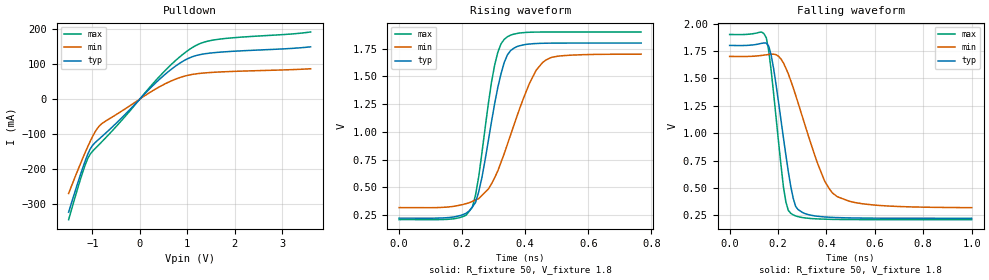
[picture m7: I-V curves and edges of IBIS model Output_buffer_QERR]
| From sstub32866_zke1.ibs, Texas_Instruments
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|   Model   Output_buffer_QERR
[Model]   Output_buffer_QERR
Model_type   Open_drain
Polarity   Non-Inverting
Vmeas  =   0.90
Cref   =   10.0p
Rref   =   1000
Vref   =   1.8
|Variable   typ   min   max
C_comp   1.120e-12   0.305e-12   1.791e-12
|Variable   typ   min   max
[Voltage range]   1.8   1.7   1.9
|Variable   typ   min   max
[Temperature range]  27   125   0.0
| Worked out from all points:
|   slope of the pulldown table from 0 to 0.27 V, typ, clamps not added: 7.15 ohm
|   rising waveform, R_fixture 50, V_fixture 1.8: 20-80 % time 61.3ps typ, 107ps min, 50.9ps max; typ from 0.223 V to 1.8 V
|   falling waveform, R_fixture 50, V_fixture 1.8: 20-80 % time 61.8ps typ, 125ps min, 48.3ps max; typ from 1.8 V to 0.223 V
[Pulldown]
|Voltage   I(typ)   I(min)   I(max)
-1.5V     -322.5mA   -269.1mA   -343.9mA
-1.25V    -215.3mA   -184.1mA   -228.5mA
-1.1V     -158.4mA   -136.7mA   -170.5mA
-1V       -132.8mA   -107.9mA   -149.4mA
-850mV    -113mA     -76.23mA   -128.7mA
-400mV    -56.04mA   -35.91mA   -63.47mA
400mV     54.51mA    33.91mA    62.36mA
700mV     88.68mA    53.85mA    103.2mA
950mV     111mA      65.61mA    132.1mA
1.25V     126.2mA    72.95mA    157.1mA
1.55V     132.1mA    76.25mA    168.3mA
3.6V      149mA      86.39mA    191.3mA
[Pullup]
|Voltage   I(typ)   I(min)   I(max)
-1.5V     0A         0A         0A
0V        0A         0A         0A
1.8V      0A         0A         0A
3.6V      0A         0A         0A
[Ramp]
|Variable   typ   min   max
dV/dt_r  0.9459/6.011e-11   0.8287/1.064e-10   1.0137/4.987e-11
dV/dt_f  0.9459/6.123e-11   0.8287/1.244e-10   1.0137/4.831e-11
R_load  =  50
[Rising Waveform]
R_fixture   =   50
V_fixture   =   1.8
V_fixture_min   =   1.7
V_fixture_max   =   1.9
C_fixture   =   0.00
|Time   V(typ)   V(min)   V(max)
0s        223.5mV    318.8mV    210.5mV
181.8ps   239.2mV    334.4mV    222.1mV
232.3ps   324.8mV    374.5mV    322.8mV
262.6ps   589.6mV    428.5mV    810.7mV
303ps     1.255V     587.5mV    1.602V
323.2ps   1.524V     726.6mV    1.793V
343.4ps   1.694V     888.8mV    1.857V
414.1ps   1.791V     1.441V     1.897V
464.6ps   1.799V     1.646V     1.9V
767.7ps   1.8V       1.7V       1.9V
[Falling Waveform]
R_fixture   =   50
V_fixture   =   1.8
V_fixture_min   =   1.7
V_fixture_max   =   1.9
C_fixture   =   0.00
|Time   V(typ)   V(min)   V(max)
0s        1.8V       1.7V       1.9V
151.5ps   1.822V     1.715V     1.87V
181.8ps   1.589V     1.72V      1.361V
222.2ps   958.1mV    1.641V     510.9mV
232.3ps   800.8mV    1.594V     373.4mV
252.5ps   514.8mV    1.479V     269mV
282.8ps   302.9mV    1.276V     238.4mV
393.9ps   235.2mV    557mV      215.3mV
444.4ps   229.8mV    421.3mV    212.8mV
1ns       223.5mV    320.4mV    210.5mV
